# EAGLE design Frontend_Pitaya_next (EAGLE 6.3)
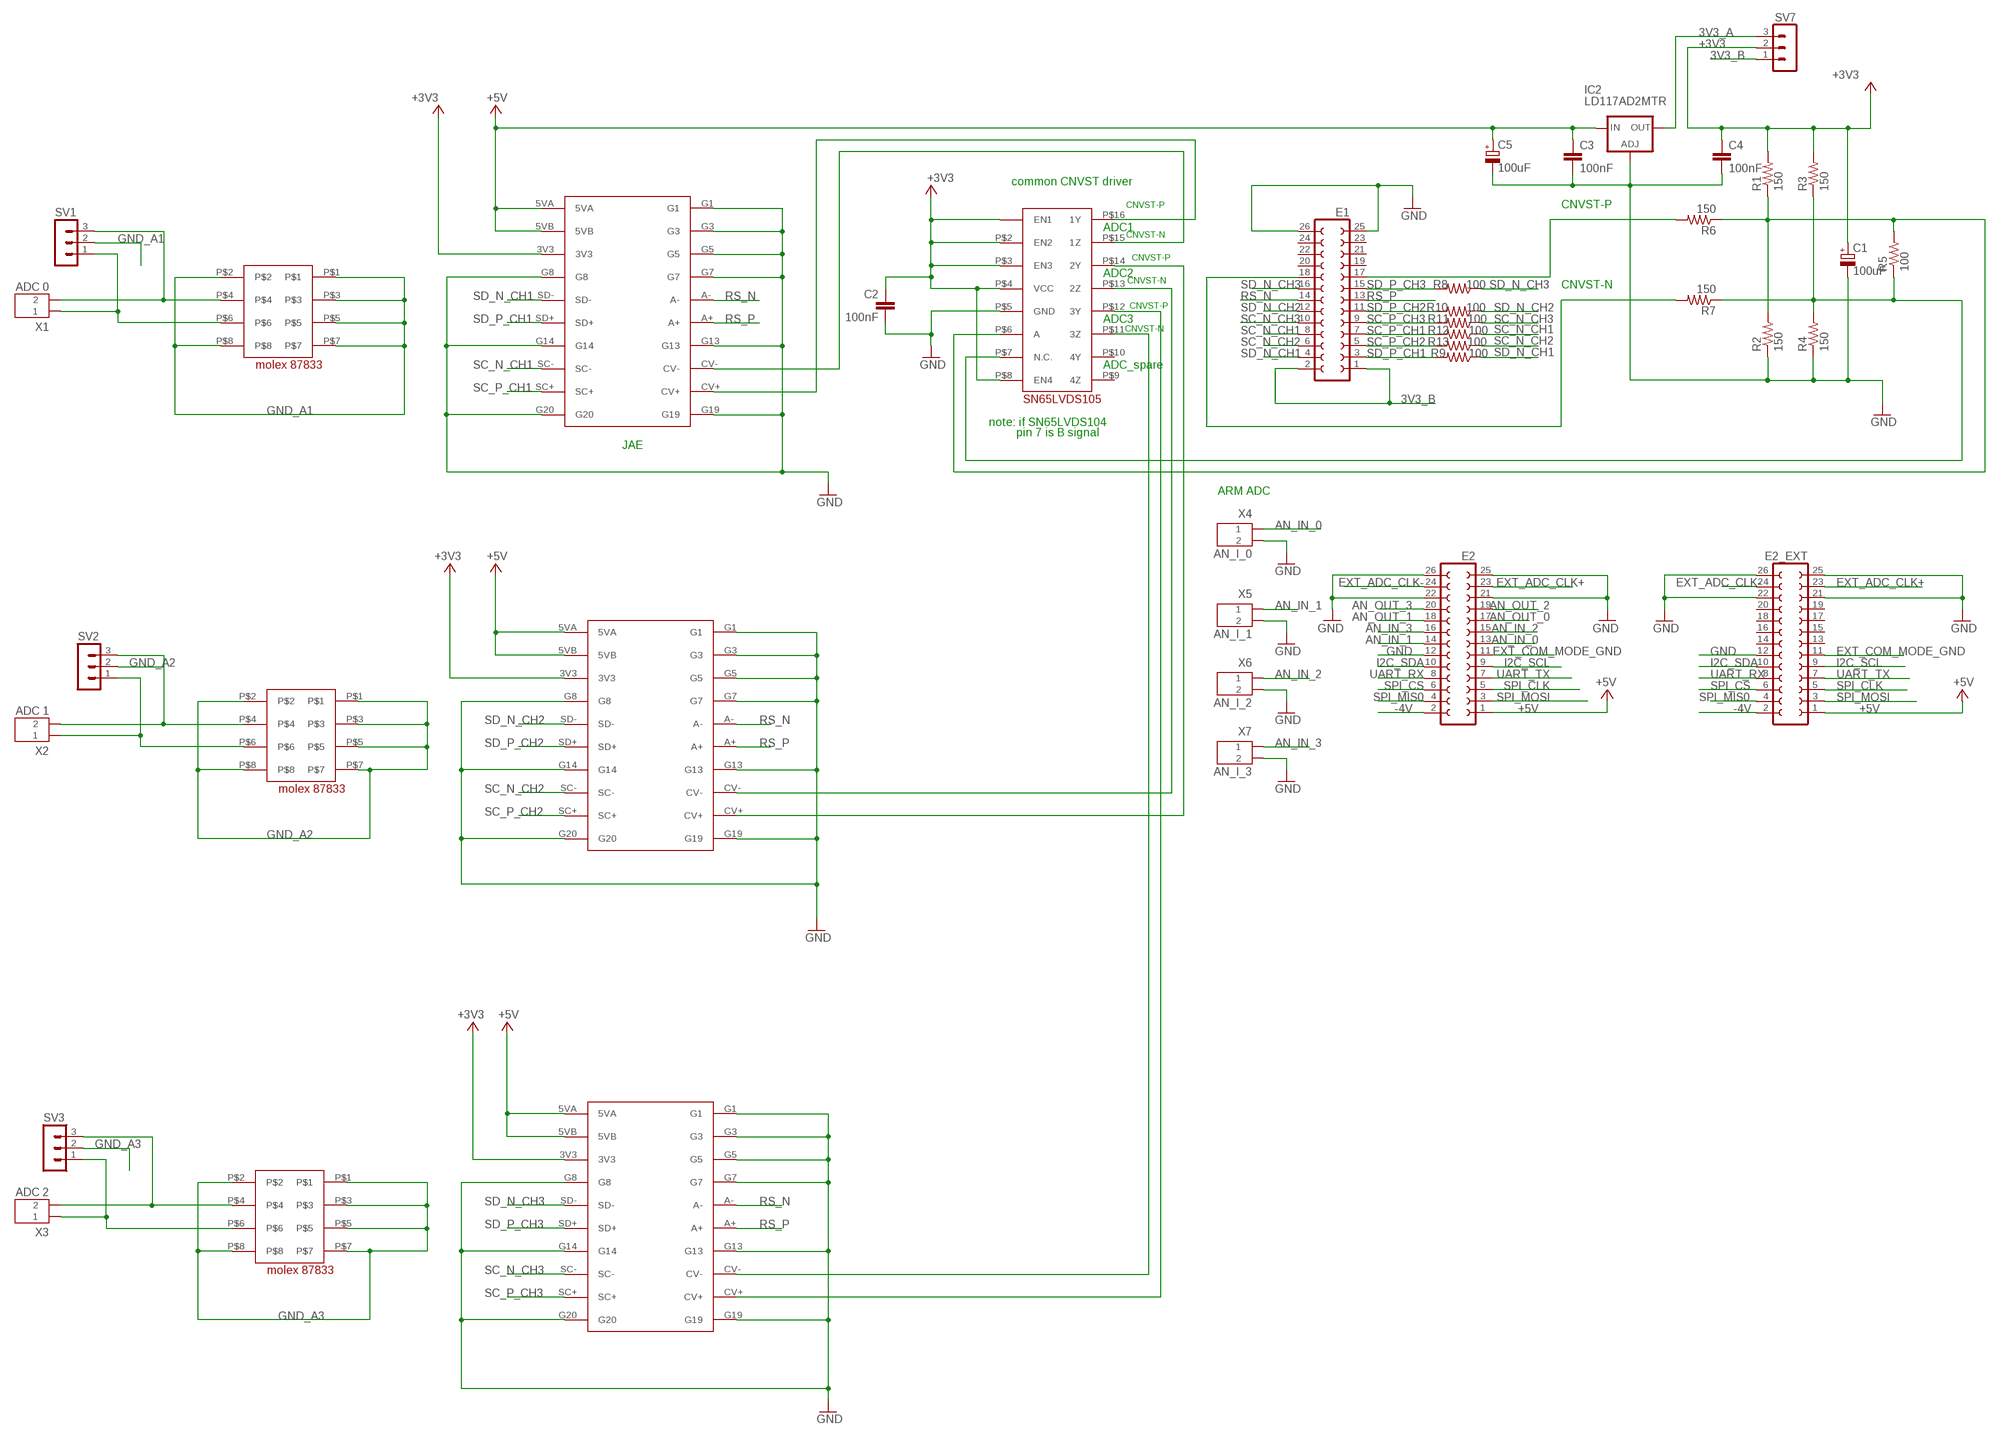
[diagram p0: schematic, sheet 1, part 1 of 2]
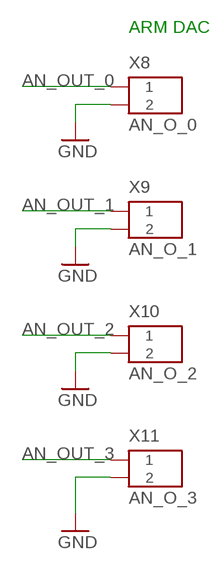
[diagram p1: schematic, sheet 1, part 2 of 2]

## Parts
C1  100uF  CPOL-EU085CS-1AR  [085CS_1AR]
C2  100nF  C-EUC0805  [C0805]
C3  100nF  C-EUC0805  [C0805]
C4  100nF  C-EUC0805  [C0805]
C5  100uF  CPOL-EU085CS-1AR  [085CS_1AR]
E1  FE13-2  [FE13-2]
E2  FE13-2  [FE13-2]
E2_EXT  FE13-2  [FE13-2]
IC2  LD117AD2MTR  [D2PACK]
R1  150  R-US_R0805  [R0805]
R2  150  R-US_R0805  [R0805]
R3  150  R-US_R0805  [R0805]
R4  150  R-US_R0805  [R0805]
R5  100  R-US_R0805  [R0805]
R6  150  R-US_R0805  [R0805]
R7  150  R-US_R0805  [R0805]
R8  100  R-US_R0805  [R0805]
R9  100  R-US_R0805  [R0805]
R10  100  R-US_R0805  [R0805]
R11  100  R-US_R0805  [R0805]
R12  100  R-US_R0805  [R0805]
R13  100  R-US_R0805  [R0805]
SV1  MA03-1  [MA03-1]
SV2  MA03-1  [MA03-1]
SV3  MA03-1  [MA03-1]
SV7  MA03-1  [MA03-1]
U$1  JAE_NEXT  [JAE_NEXT]
U$2  MOLEX87833_NEXT  [MOLEX87833NEXT]
U$3  SN65LVDS105  [SN65LVDS105]
U$4  MOLEX87833_NEXT  [MOLEX87833NEXT]
U$5  JAE_NEXT  [JAE_NEXT]
U$6  MOLEX87833_NEXT  [MOLEX87833NEXT]
U$7  JAE_NEXT  [JAE_NEXT]
X1  ADC 0  EZG-00-302  [EZG-00-302]
X2  ADC 1  EZG-00-302  [EZG-00-302]
X3  ADC 2  EZG-00-302  [EZG-00-302]
X4  AN_I_0  EZG-00-302  [EZG-00-302]
X5  AN_I_1  EZG-00-302  [EZG-00-302]
X6  AN_I_2  EZG-00-302  [EZG-00-302]
X7  AN_I_3  EZG-00-302  [EZG-00-302]
X8  AN_O_0  EZG-00-302  [EZG-00-302]
X9  AN_O_1  EZG-00-302  [EZG-00-302]
X10  AN_O_2  EZG-00-302  [EZG-00-302]
X11  AN_O_3  EZG-00-302  [EZG-00-302]

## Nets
3V3_A: IC2.2(OUT) SV7.3
3V3_B: E1.1 E1.2 SV7.1
+3V3: C1.+ C2.1 C4.1 R1.2 R3.2 SV7.2 U$1.3V3 U$3.P$1(EN1) U$3.P$2(EN2) U$3.P$3(EN3) U$3.P$4(VCC) U$3.P$8(EN4) U$5.3V3 U$7.3V3
+5V: C3.1 C5.+ E2.1 E2_EXT.1 IC2.3(IN) U$1.5VA U$1.5VB U$5.5VA U$5.5VB U$7.5VA U$7.5VB
-4V: E2.2 E2_EXT.2
AN_IN_0: E2.13 X4.1
AN_IN_1: E2.14 X5.1
AN_IN_2: E2.15 X6.1
AN_IN_3: E2.16 X7.1
AN_OUT_0: E2.17 X8.1
AN_OUT_1: E2.18 X9.1
AN_OUT_2: E2.19 X10.1
AN_OUT_3: E2.20 X11.1
EXT_ADC_CLK+: E2.23 E2_EXT.23
EXT_ADC_CLK-: E2.24 E2_EXT.24
EXT_COM_MODE_GND: E2.11 E2_EXT.11
GND: C1.- C2.2 C3.2 C4.2 C5.- E1.25 E1.26 E2.12 E2.21 E2.22 E2.25 E2.26 E2_EXT.12 E2_EXT.21 E2_EXT.22 E2_EXT.25 E2_EXT.26 IC2.1(ADJ) R2.1 R4.1 U$1.G1 U$1.G3 U$1.G5 U$1.G7 U$1.G8 U$1.G13 U$1.G14 U$1.G19 U$1.G20 U$3.P$5(GND) U$5.G1 U$5.G3 U$5.G5 U$5.G7 U$5.G8 U$5.G13 U$5.G14 U$5.G19 U$5.G20 U$7.G1 U$7.G3 U$7.G5 U$7.G7 U$7.G8 U$7.G13 U$7.G14 U$7.G19 U$7.G20 X4.2 X5.2 X6.2 X7.2 X8.2 X9.2 X10.2 X11.2
GND_A1: SV1.2 U$6.P$1 U$6.P$2 U$6.P$3 U$6.P$5 U$6.P$7 U$6.P$8
GND_A2: SV2.2 U$4.P$1 U$4.P$2 U$4.P$3 U$4.P$5 U$4.P$7 U$4.P$8
GND_A3: SV3.2 U$2.P$1 U$2.P$2 U$2.P$3 U$2.P$5 U$2.P$7 U$2.P$8
I2C_SCL: E2.9 E2_EXT.9
I2C_SDA: E2.10 E2_EXT.10
N$1: SV1.3 U$6.P$4 X1.2
N$9: E1.17 R6.2
N$11: E1.18 R7.2
N$24: SV1.1 U$6.P$6 X1.1
N$27: SV2.3 U$4.P$4 X2.2
N$30: U$3.P$16(1Y) U$7.CV+
N$31: U$3.P$15(1Z) U$7.CV-
N$32: SV2.1 U$4.P$6 X2.1
N$33: SV3.3 U$2.P$4 X3.2
N$34: R3.1 R4.2 R5.1 R7.1 U$3.P$7(N.C.)
N$35: U$3.P$14(2Y) U$5.CV+
N$36: SV3.1 U$2.P$6 X3.1
N$37: U$3.P$13(2Z) U$5.CV-
N$38: U$1.CV+ U$3.P$12(3Y)
N$39: U$1.CV- U$3.P$11(3Z)
N$40: R1.1 R2.2 R5.2 R6.1 U$3.P$6(A)
RS_N: E1.14 U$1.A- U$5.A- U$7.A-
RS_P: E1.13 U$1.A+ U$5.A+ U$7.A+
SC_N_CH1: E1.8 R12.1 U$7.SC-
SC_N_CH2: E1.6 R13.1 U$5.SC-
SC_N_CH3: E1.10 R11.1 U$1.SC-
SC_P_CH1: E1.7 R12.2 U$7.SC+
SC_P_CH2: E1.5 R13.2 U$5.SC+
SC_P_CH3: E1.9 R11.2 U$1.SC+
SD_N_CH1: E1.4 R9.1 U$7.SD-
SD_N_CH2: E1.12 R10.1 U$5.SD-
SD_N_CH3: E1.16 R8.1 U$1.SD-
SD_P_CH1: E1.3 R9.2 U$7.SD+
SD_P_CH2: E1.11 R10.2 U$5.SD+
SD_P_CH3: E1.15 R8.2 U$1.SD+
SPI_CLK: E2.5 E2_EXT.5
SPI_CS: E2.6 E2_EXT.6
SPI_MIS0: E2.4 E2_EXT.4
SPI_MOSI: E2.3 E2_EXT.3
UART_RX: E2.8 E2_EXT.8
UART_TX: E2.7 E2_EXT.7
Unconnected: E1.19 E1.20 E1.21 E1.22 E1.23 E1.24 E2_EXT.13 E2_EXT.14 E2_EXT.15 E2_EXT.16 E2_EXT.17 E2_EXT.18 E2_EXT.19 E2_EXT.20 U$3.P$9(4Z) U$3.P$10(4Y)

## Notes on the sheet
- common CNVST driver
- CNVST-P | CNVST-P
- ADC1
- CNVST-N
- CNVST-P
- ADC2
- CNVST-N
- CNVST-N
- CNVST-P
- ADC3
- CNVST-N
- ADC_spare
- note: if SN65LVDS104
- pin 7 is B signal
- JAE
- ARM DAC
- ARM ADC

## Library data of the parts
C1 C5 = resistor:CPOL-EU: POLARIZED CAPACITOR, European symbol
C2-C4 = resistor:C-EU: CAPACITOR, European symbol
E1 E2 E2_EXT = con-lsta:FE13-2: FEMALE HEADER; OC_FARNELL: unknown; OC_NEWARK: unknown
IC2 = v-reg:LD117A?*: Low drop fixed and adjustable positive voltage regulators 1 A Source: http://www.st.com/stonline/products/literature/ds/7194/ld1117axx.pdf
R1-R13 = resistor:R-US_: RESISTOR, American symbol
SV1-SV3 SV7 = con-lstb:MA03-1: PIN HEADER; OC_FARNELL: unknown; OC_NEWARK: unknown
U$1 U$5 U$7 = JAE_pad_extend:JAE_NEXT: JAE_Connector Next
U$2 U$4 U$6 = molex 87833 next:MOLEX87833_NEXT: Molex 87833 next
U$3 = SN65LVDS105:SN65LVDS105
X1-X11 = con-lemo:EZG-?-302: LEMO Connector; OC_FARNELL: unknown; OC_NEWARK: unknown

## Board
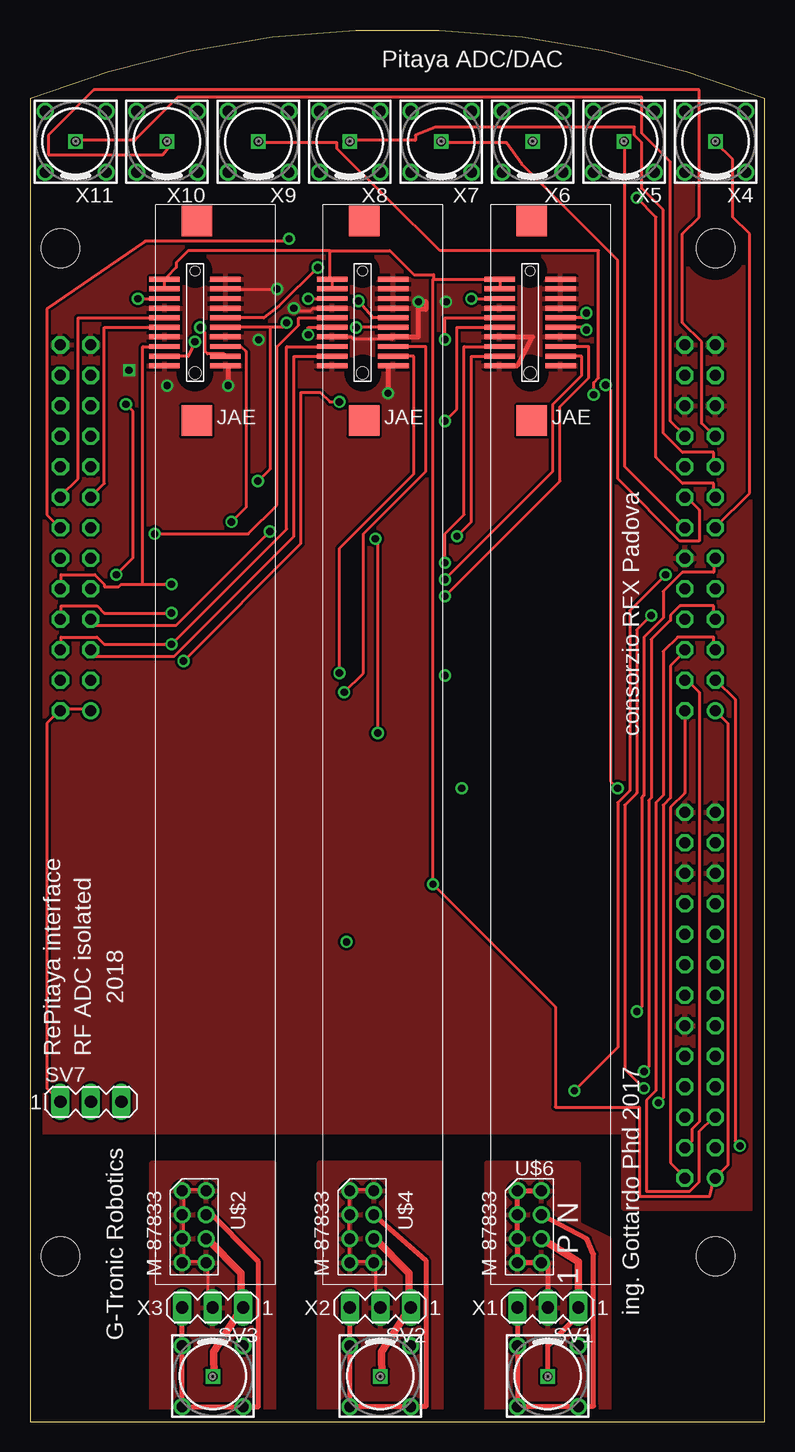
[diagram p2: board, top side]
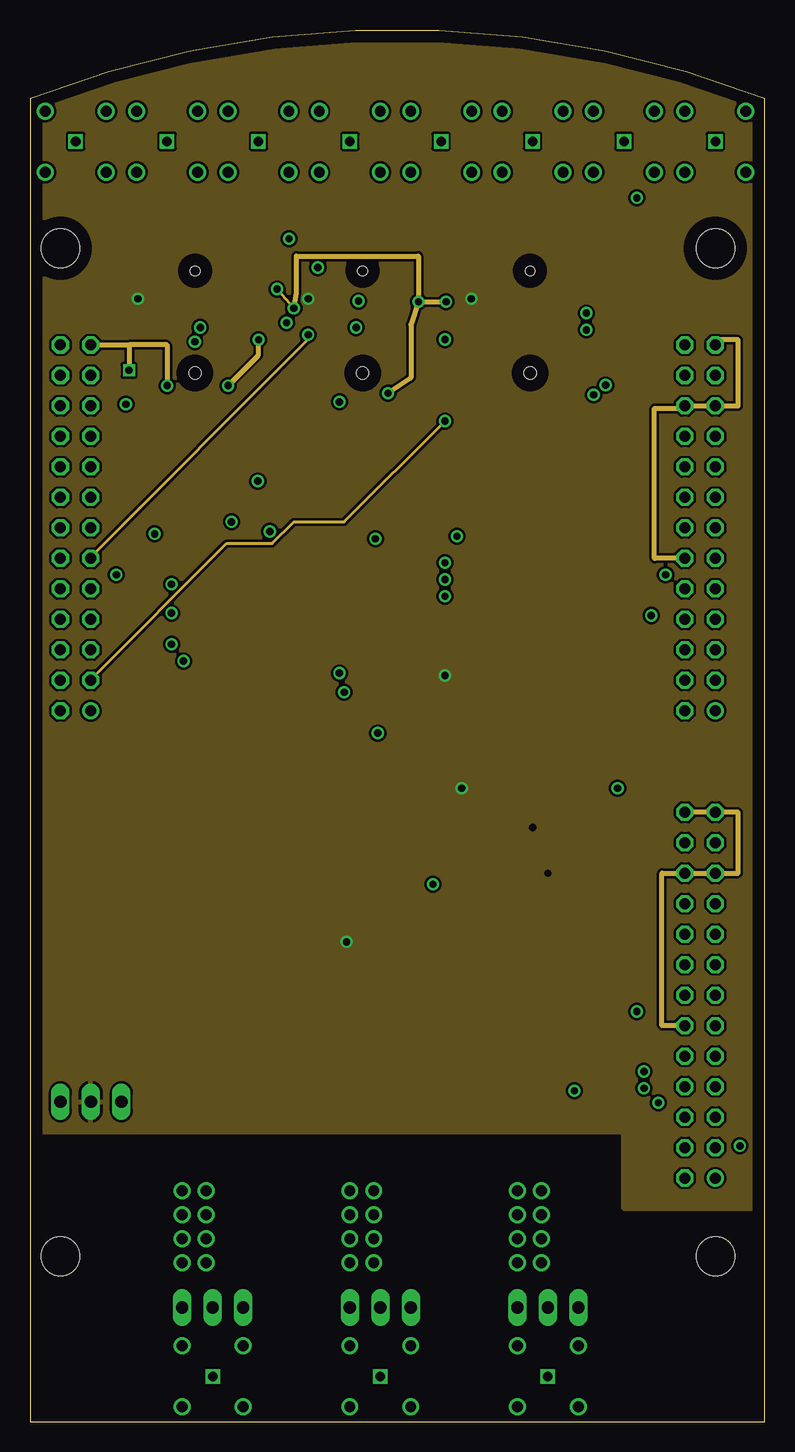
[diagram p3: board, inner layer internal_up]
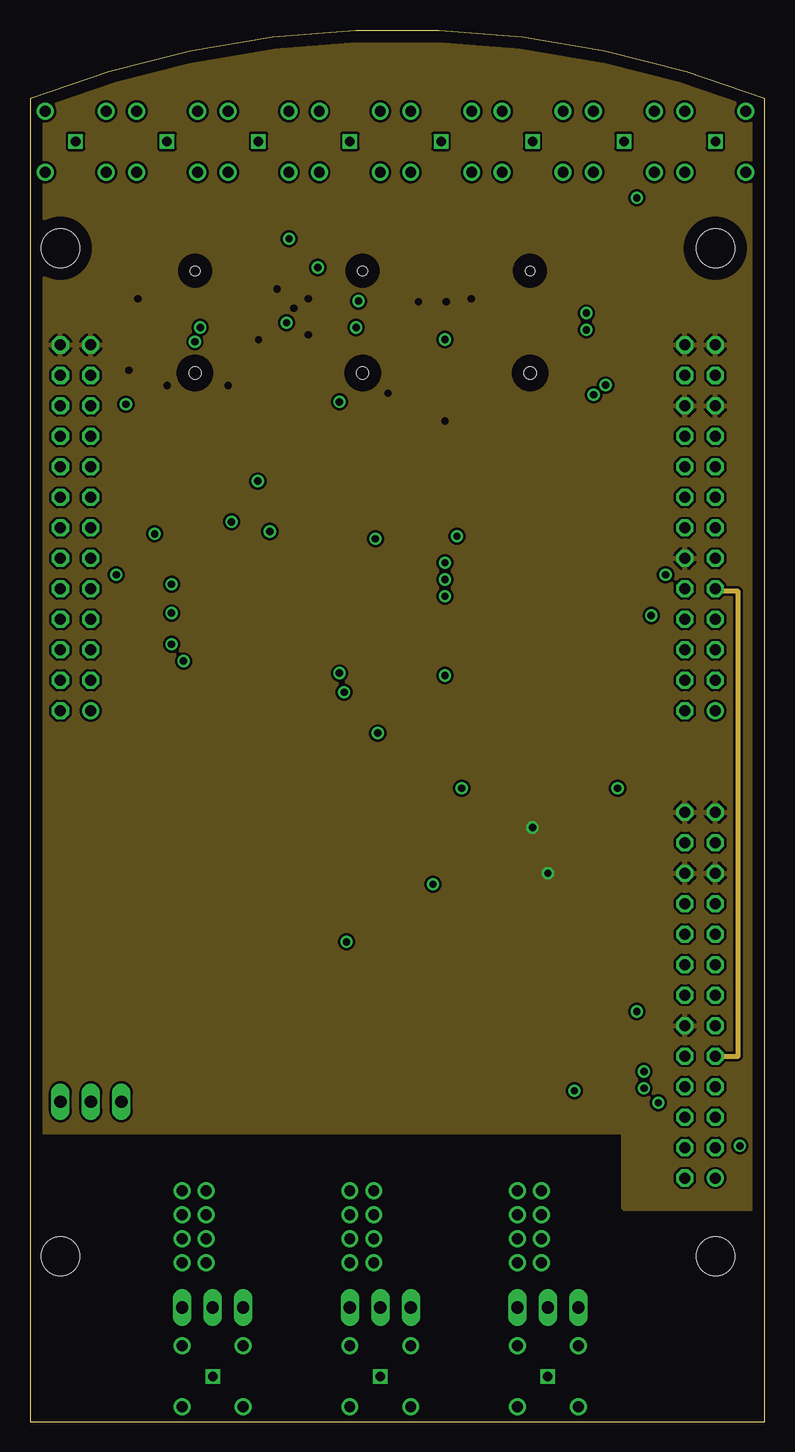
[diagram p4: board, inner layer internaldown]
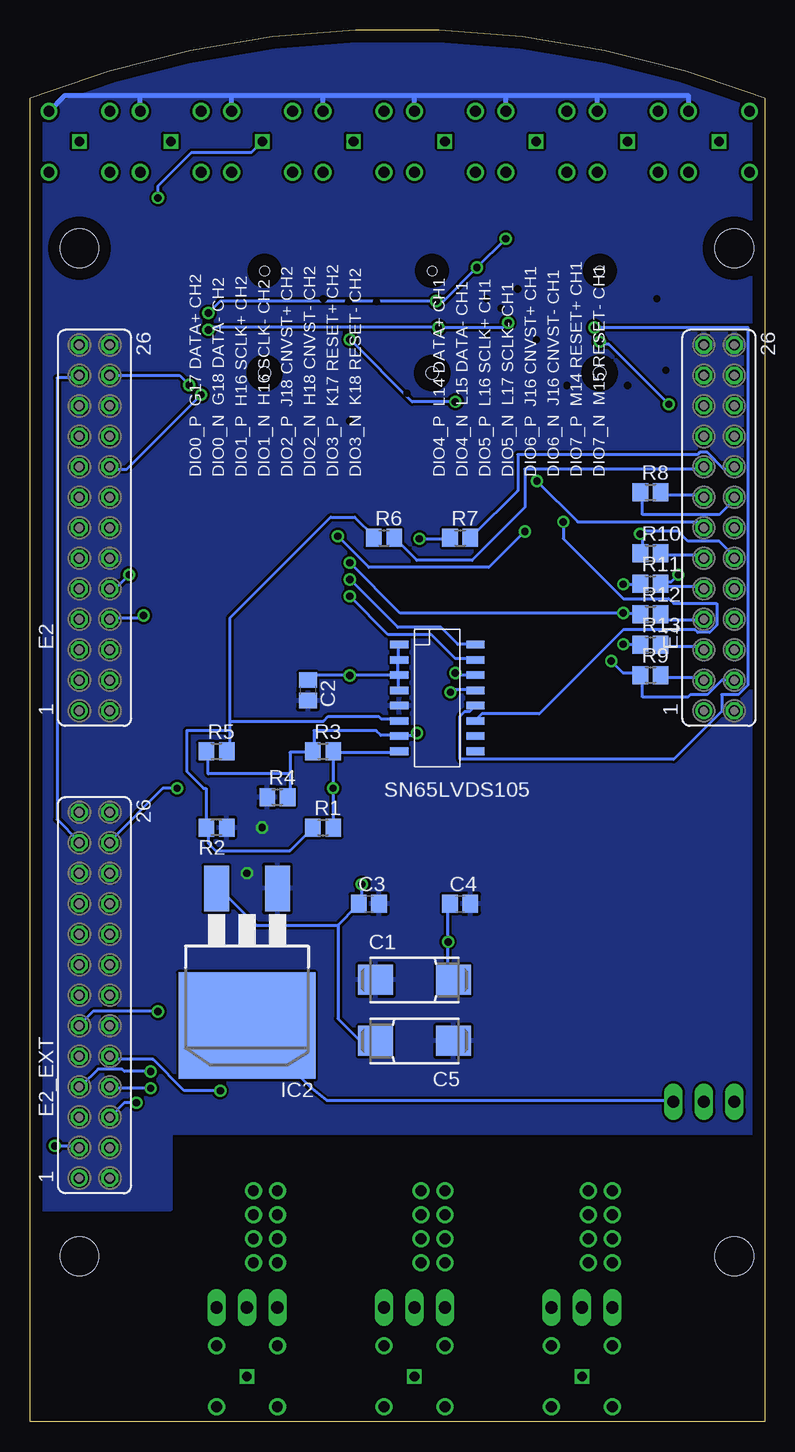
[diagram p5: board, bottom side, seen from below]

Size 61.27 x 115.99 mm. Coordinates in mm from the lower left corner, seen from the top.
Outline: 0,0 61.27,0 61.27,110.32 arc42 0,110.32 0,0
Copper layers ((1*2)+(15*16)): Top 0.035mm / dielectric 1.5mm / internal_up 0.035mm / dielectric 0.15mm / internaldown 0.035mm / dielectric 0.2mm / Bottom 0.035mm
Design rules "default *": minimum track width 10mil, minimum drill 24mil, track to track 8mil, track to pad 8mil, pad to pad 8mil, via to via 8mil, smd to smd 8mil, copper to edge 40mil, drill to drill 8mil, minimum pad ring 10mil, minimum via ring 8mil, stop-mask expansion 4mil, vias tented up to drill 0mil, thermal gap 10mil
Holes 3.2 mm at 2.54,97.8 57.15,97.8 2.54,13.8 57.15,13.8

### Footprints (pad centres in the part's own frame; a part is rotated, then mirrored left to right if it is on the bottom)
085CS_1AR = smd 2.9 x 2.5: + 3.25,0; - -3.25,0
C0805 = smd 1.3 x 1.5: 1 -0.85,0; 2 0.85,0
FE13-2 = drill 0.914: 1 -15.24,1.27 | drill 0.914 octagon: 2 -15.24,-1.27; 3 -12.7,1.27; 4 -12.7,-1.27; 5 -10.16,1.27; 6 -10.16,-1.27; 7 -7.62,1.27; 8 -7.62,-1.27; 9 -5.08,1.27; 10 -5.08,-1.27; 11 -2.54,1.27; 12 -2.54,-1.27; 13 0,1.27; 14 0,-1.27; 15 2.54,1.27; 16 2.54,-1.27; 17 5.08,1.27; 18 5.08,-1.27; 19 7.62,1.27; 20 7.62,-1.27; 21 10.16,1.27; 22 10.16,-1.27; 23 12.7,1.27; 24 12.7,-1.27; 25 15.24,1.27; 26 15.24,-1.27
D2PACK = smd 2.083 x 3.81: 1 -2.54,-8.89; 3 2.54,-8.89 | smd 11.43 x 8.89: 2 0,2.54
R0805 = smd 1.3 x 1.5: 1 -0.85,0; 2 0.85,0
MA03-1 = drill 1.016 long: 1 -2.54,0; 2 0,0; 3 2.54,0
JAE_NEXT = smd 2.54 x 0.406: 3V3 -2.748,1.155; 5VA -2.748,2.755; 5VB -2.748,1.955; A+ 2.337,-1.245; A- 2.337,-0.445; CV+ 2.337,-3.645; CV- 2.337,-2.845; G1 2.337,2.755; G3 2.337,1.955; G5 2.337,1.155; G7 2.337,0.355; G8 -2.748,0.355; G13 2.337,-2.045; G14 -2.748,-2.045; G19 2.337,-4.445; G20 -2.748,-4.445; SC+ -2.748,-3.645; SC- -2.748,-2.845; SD+ -2.748,-1.245; SD- -2.748,-0.445 | smd 2.54 x 2.54: P$1 -0.071,7.62; P$2 -0.071,-9.017 | hole 0.8: -0.205,3.455 | hole 1: -0.205,-5.045
MOLEX87833NEXT = drill 0.9: P$1 -1.27,1.27; P$2 -1.27,3.27; P$3 0.73,1.27; P$4 0.73,3.27; P$5 2.73,1.27; P$6 2.73,3.27; P$7 4.73,1.27; P$8 4.73,3.27
SN65LVDS105 = smd 1.524 x 0.635: P$1 -2.54,8.89; P$2 -2.54,7.62; P$3 -2.54,6.35; P$4 -2.54,5.08; P$5 -2.54,3.81; P$6 -2.54,2.54; P$7 -2.54,1.27; P$8 -2.54,0; P$9 3.81,0; P$10 3.81,1.27; P$11 3.81,2.54; P$12 3.81,3.81; P$13 3.81,5.08; P$14 3.81,6.35; P$15 3.81,7.62; P$16 3.81,8.89
EZG-00-302 = drill 0.6 pad 1: 1 0,-0.035; 2 -2.54,-2.505 | drill 0.9 pad 1.2: M1 -2.54,2.54; M2 2.54,2.54; M3 2.54,-2.54; M4 -2.54,-2.54

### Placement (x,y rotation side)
C1  29.21,36.83 0 bottom
C2  38.1,60.96 270 bottom
C3  33.02,43.18 0 bottom
C4  25.4,43.18 0 bottom
C5  29.21,31.75 180 bottom
E1  3.81,74.5 90 bottom
E2  55.88,74.5 90 bottom
E2_EXT  55.88,35.56 90 bottom
IC2  43.18,35.56 180 bottom
R1  36.83,49.53 0 bottom
R2  45.72,49.53 180 bottom
R3  36.83,55.88 0 bottom
R4  40.64,52.07 0 bottom
R5  45.72,55.88 0 bottom
R6  31.75,73.66 0 bottom
R7  25.4,73.66 0 bottom
R8  9.53,77.47 0 bottom
R9  9.53,62.23 0 bottom
R10  9.53,72.39 0 bottom
R11  9.53,69.85 0 bottom
R12  9.53,67.31 0 bottom
R13  9.53,64.77 0 bottom
SV1  43.18,9.53 180 top
SV2  29.21,9.53 180 top
SV3  15.24,9.53 180 top
SV7  5.08,26.67 0 top
U$1  13.97,92.46 0 top
U$2  11.43,18 270 top
U$3  27.94,55.88 0 bottom
U$4  25.4,18 270 top
U$5  27.94,92.46 0 top
U$6  39.37,18 270 top
U$7  41.91,92.46 0 top
X1  43.18,3.81 0 top
X2  29.21,3.81 0 top
X3  15.24,3.81 0 top
X4  57.15,106.68 180 top
X5  49.53,106.68 180 top
X6  41.91,106.68 180 top
X7  34.29,106.68 180 top
X8  26.67,106.68 180 top
X9  19.05,106.68 180 top
X10  11.43,106.68 180 top
X11  3.81,106.68 180 top

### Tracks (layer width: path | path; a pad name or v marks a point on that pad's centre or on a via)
3V3_A
  Bottom 0.254: SV7.3 7.8,26.8 36.53,26.8 37.8,27.8 43,33 IC2.2
3V3_B
  Top 0.254: E1.1 5,59.4 2.6,59.4 E1.2 2.4,59.2 1.4,58.2 1.4,27.8 2.4,26.8 SV7.1
+3V3  (via drill 0.61, 0.61 layers 1-2)
  Top 0.254: v9,93.6 11.2,93.6 U$1.3V3 | v23.2,93.6 25,93.6 U$5.3V3 | v36.8,93.6 39,93.6 U$7.3V3
  Bottom 0.254: R1.2 36,49.6 v36,52.8 36,55.8 R3.2 35.8,55.8 30.6,55.8 U$3.P$8 | U$3.P$1 30.6,64.6 30.6,63.6 U$3.P$2 30.6,63.4 30.6,62.4 U$3.P$3 30.6,62.2 | 30.6,62.2 v34.6,62.2 37.8,62.2 38,62 C2.1 | 30.6,62.2 30.6,61 U$3.P$4 | C4.1 26.4,43 v26.4,40 26.4,37 26,37 C1.+
  pour internal_up: -11.43,121.92 69.85,121.92 69.85,17.78 49.53,17.78 49.53,24.13 -11.43,24.13
+5V  (via drill 0.61)
  Top 0.254: E2.1 57.2,59.2 58.2,58.2 58.2,21.4 57.2,20.4 E2_EXT.1 57,20.2 56.67,18.8 50.8,18.8 50.8,26.22 43.8,26.22 43.8,34.6 v33.6,44.8 33.6,95.2 33.66,95.2 | U$7.5VB 39.2,94.6 39.2,95.2 U$7.5VA 39,95.2 33.66,95.2 | U$1.5VB 11.2,94.6 11.2,95.2 U$1.5VA 11.4,95.4 12.2,96.2 12.2,96.6 13.2,97.6 25,97.6 | U$5.5VB 25.2,94.6 U$5.5VA 25,95.4 25,97.6 | 33.66,95.2 33.66,95.6 32,95.6 30,97.6 25,97.6
  Bottom 0.254: 35.6,41.4 34,43 C3.1 33.8,43.2 33.6,43.2 v33.6,44.8 | 35.6,41.4 42.4,41.4 45.4,44.4 45.6,44.4 IC2.3 | 35.6,41.4 35.6,33.61 33.87,31.88 C5.+
-4V
  Top 0.254: E2_EXT.2 54.6,20.4 53.4,21.6 53.4,51.2 54.6,52.4 54.6,59.2 E2.2
AN_IN_0
  Top 0.254: X4.1 57.2,106.6 58.6,105.2 58.6,100.4 60,99 60,77.4 57.2,74.6 E2.13
AN_IN_1
  Top 0.254: X5.1 49.6,106.6 49.6,79.6 54.6,74.6 E2.14
AN_IN_2  (via drill 0.61)
  Top 0.254: v50.6,102 52.2,100.4 52.2,80.4 54.4,78.2 57,78.2 57,77.2 E2.15
  Bottom 0.254: v50.6,102 50.6,103 47.8,105.8 42.8,105.8 42,106.6 X6.1
AN_IN_3
  Top 0.254: X7.1 34.4,106.6 39.73,106.6 41,104.8 49,96.8 49,78.6 54.2,73.4 55.8,73.4 55.8,76 54.8,77 E2.16
AN_OUT_0
  Top 0.254: X8.1 26.8,106.8 32.13,106.8 32.13,107.2 33.8,107.9 50.4,107.9 50.4,107.2 51,106.6 51,102.8 52.8,101 52.8,82.4 54.4,80.8 57,80.8 57,79.6 E2.17
AN_OUT_1  (via drill 0.61)
  Top 0.254: v47,85.6 47,86.6 47.4,87 47.4,97.6 34.2,97.6 25.6,106.1 25.6,106.6 19.2,106.6 X9.1
  Bottom 0.254: v47,85.6 53.2,79.4 54.6,79.4 E2.18
AN_OUT_2
  Top 0.254: X10.1 11.4,106.6 11.87,106.6 11.07,105.6 1.53,105.6 1.53,107.2 5.33,111 55.8,111 55.8,100.4 54.4,99 54.4,91.6 56,90 56,83.2 57,82.2 E2.19
AN_OUT_3
  Top 0.254: X11.1 4,106.8 8.73,106.8 12.33,110.4 51,110.4 51,107.4 53.4,105 53.4,83.4 54.6,82.2 E2.20
EXT_ADC_CLK+
  Bottom 0.254: E2_EXT.23 57.2,48.4 59,50.2 59,87 57.4,87 57.2,87.2 E2.23
EXT_ADC_CLK-  (via drill 0.61)
  Top 0.254: v49,52.8 48.4,53.4 48.4,86 v48,86.4
  Bottom 0.254: v49,52.8 50.2,52.8 54.6,48.4 E2_EXT.24 | v48,86.4 48.8,87.2 E2.24
EXT_COM_MODE_GND  (via drill 0.61)
  Top 0.254: v50.6,34.2 51,34.6 51,52 51.2,52.2 51.2,65.4 52.8,67 52.8,69.2 54.4,70.8 57,70.8 57,71.8 E2.11
  Bottom 0.254: v50.6,34.2 56,34.2 57,33.2 E2_EXT.11
GND  (via drill 0.6 layers 1-2, 0.6 layers 15-16, 0.61 layers 1-2)
  Top 0.254: U$5.G14 26.8,90.4 27,90.2 30.2,90.2 30.2,90.4 U$5.G13 | v22,92.8 22,92.6 23.4,92.6 23.6,92.8 25,92.8 U$5.G8 | v20.6,94.4 16.4,94.4 U$1.G3
  Top 0.406: U$5.G19 29.84,88.01 v29.84,85.72 | U$5.G13 32.38,90.41 v32.38,93.34 | v32.38,93.34 33.02,93.34 33.02,92.71 32.38,92.71 v32.38,93.34 | U$7.G14 41.91,90.41 40.64,88.01 U$7.G20 | U$1.G19 16.51,88.01 v16.51,86.36
  internal_up 0.254: v20.6,94.4 v22,92.8 | 34.8,93.2 v34.7,93.34
  internal_up 0.406: E2.12 52.07,71.96 52.07,84.45 54.61,84.45 E2.22 E2.21 59.05,84.66 59.05,90.17 57.15,90.17 E2.25 | E2_EXT.12 52.7,33.02 52.7,45.72 E2_EXT.22 E2_EXT.21 59.05,45.72 59.05,50.8 E2_EXT.25 E2_EXT.26 | E1.25 8.26,89.74 | v11.43,86.36 11.43,89.74 8.26,89.74 | v32.38,93.34 v34.7,93.34 | v32.38,93.34 31.75,91.44 31.75,87 v29.84,85.72 | 22.02,92.81 22.23,94.08 22.23,97.16 32.38,97.16 v32.38,93.34 | 8.26,89.74 v8.26,87.63 | v16.51,86.36 19.05,88.9 v19.05,90.17
  Bottom 0.406: X11.2 6.35,110.49 13.97,110.49 | X10.2 13.97,110.49 | 13.97,110.49 21.59,110.49 | X9.2 21.59,110.49 | 21.59,110.49 29.21,110.49 | X8.2 29.21,110.49 | 29.21,110.49 36.83,110.49 | X7.2 36.83,110.49 | 36.83,110.49 44.45,110.49 | X6.2 44.45,110.49 | 44.45,110.49 52.07,110.49 | X5.2 52.07,110.49 | 52.07,110.49 58.42,110.49 X4.2
  other vias: 41.91,49.53 43.18,45.72
  pour Bottom: -6.35,118.11 64.77,118.11 64.77,17.78 49.53,17.78 49.53,24.13 -6.35,24.13
  pour Top: -8.89,119.38 67.31,119.38 68.58,17.78 49.53,17.78 49.53,24.13 -7.62,24.13
  pour internaldown: -12.7,123.19 73.66,123.19 73.66,17.78 49.53,17.78 49.53,24.13 -12.7,24.13
GND_A1
  Top 0.406: SV1.2 43.18,13.27 U$6.P$8 U$6.P$7 U$6.P$5 U$6.P$3 U$6.P$1 U$6.P$2
  pour Top: 38.1,21.59 45.72,21.59 45.72,16.51 48.26,15.24 48.26,-1.27 38.1,-1.27
GND_A2
  Top 0.254: U$4.P$2 28.6,19.4 26.8,19.4 U$4.P$1 26.6,19.2 26.6,17.4 U$4.P$3 26.6,17.2 26.6,15.4 U$4.P$5 26.6,15.2 26.6,13.4 U$4.P$7 26.8,13.4 28.6,13.4 U$4.P$8 28.8,13.2 28.8,10 29.2,9.6 SV2.2
  pour Top: 24.13,21.59 34.29,21.59 34.29,-1.27 24.13,-1.27
GND_A3
  Top 0.254: U$2.P$2 14.6,19.4 12.8,19.4 U$2.P$1 12.8,19.2 12.8,17.4 U$2.P$3 12.8,17.2 12.8,15.4 U$2.P$5 12.8,15.2 12.8,13.4 | 12.8,13.4 14.6,13.4 U$2.P$8 14.8,13.2 14.8,10 15.2,9.6 SV3.2 | 12.8,13.4 U$2.P$7
  pour Top: 10.16,21.59 20.32,21.59 20.32,-1.27 10.16,-1.27
I2C_SCL
  internaldown 0.406: E2_EXT.9 59.05,30.48 59.05,69.22 57.15,69.22 E2.9
I2C_SDA  (via drill 0.61)
  Top 0.254: v45.4,27.6 49,31.2 49,51.6 50,52.6 50,67.6 v53,70.6
  Bottom 0.254: v45.4,27.6 48.4,27.6 51,30.2 54.4,30.2 54.6,30.4 E2_EXT.10 | v53,70.6 54,69.6 54.6,69.6 E2.10
N$1
  Top 0.406: SV1.3 X1.2 | 40.64,1.27 X1.2 | X1.2 46.99,1.3 46.99,13.97 46.45,15.24 U$6.P$4
N$2  (via drill 0.8)
  other vias: 29.21,3.78
N$3  (via drill 0.8)
  other vias: 15.24,3.78
N$4  (via drill 0.8)
  other vias: 3.81,106.7
N$5  (via drill 0.8)
  other vias: 11.43,106.7
N$6  (via drill 0.8)
  other vias: 19.05,106.7
N$7  (via drill 0.8)
  other vias: 26.67,106.7
N$8  (via drill 0.8)
  other vias: 34.29,106.7
N$9
  Bottom 0.254: R6.2 30.8,73.6 29,71.8 24.4,71.8 20,76.2 20,79.4 5.2,79.4 E1.17
N$10  (via drill 0.8)
  other vias: 41.91,106.7
N$11
  Bottom 0.254: R7.2 24.4,73.8 20.6,77.6 20.6,80.6 5.6,80.6 5.4,80.8 4.8,80.8 3.4,79.4 2.6,79.4 E1.18
N$12  (via drill 0.8)
  other vias: 49.53,106.7
N$13  (via drill 0.8)
  other vias: 57.15,106.7
N$24  (via drill 0.8)
  Top 0.406: X1.1 v43.18,3.78 43.18,6.35 45.72,8.89 SV1.1 | 42.64,15.24 U$6.P$6
  Top 0.61: SV1.1 45.72,13.34 42.64,15.24
N$27
  Top 0.406: U$4.P$4 33.02,13.46 33.02,1.27 26.67,1.27 X2.2 SV2.3
N$30  (via drill 0.61)
  Top 0.254: v34.6,70.2 43.6,79.2 43.6,84.8 46,87.2 46,88.8 44.4,88.8 U$7.CV+
  Bottom 0.254: v34.6,70.2 30.6,66.2 27,66.2 25.6,64.8 24.2,64.8 U$3.P$16
N$31  (via drill 0.61)
  Top 0.254: v34.6,68.8 44.2,78.4 44.2,84.6 46.6,87 46.6,89.6 44.4,89.6 U$7.CV-
  Bottom 0.254: v34.6,68.8 31.4,65.6 27.8,65.6 25.8,63.6 24.2,63.6 U$3.P$15
N$32
  Top 0.254: 29.4,3.8 X2.1 | 31.6,9.4 SV2.1 31.6,9.6 | 28.8,15.2 U$4.P$6
  Top 0.61: 29.4,3.8 29.33,5 29.33,5.86 31.6,9.4 | 28.8,15.2 31.6,12.4 31.6,9.6
N$33
  Top 0.406: U$2.P$4 14.7,17.78 19.05,13.34 19.05,1.27 12.7,1.27 X3.2 SV3.3
N$34  (via drill 0.61)
  Top 0.254: v28.8,73.6 29,73.4 v29,57.4
  Bottom 0.254: 39.6,54 39.6,55.8 37.8,55.8 R3.1 37.6,56 37.6,57.6 32.4,57.6 32,57.2 30.6,57.2 U$3.P$7 30.4,57.2 29.2,57.2 v29,57.4 | 39.6,54 39.6,52.2 R4.2 | 39.6,54 46.4,54 46.4,55.8 R5.1 | v28.8,73.6 26.4,73.6 R7.1
N$35  (via drill 0.61)
  Top 0.254: v25.8,62.4 25.8,72.8 32,79 32,88.8 30.4,88.8 U$5.CV+
  Bottom 0.254: v25.8,62.4 25.6,62.2 24.2,62.2 U$3.P$14
N$36
  Top 0.254: 15.4,3.8 X3.1 | 17.6,9.4 SV3.1 17.6,9.6 | 14.8,15.2 U$2.P$6
  Top 0.61: 15.4,3.8 15.33,5 15.33,5.86 17.6,9.4 | 14.8,15.2 17.6,12.4 17.6,9.6
N$37  (via drill 0.61)
  Top 0.254: v26.2,60.8 27.8,62.4 27.8,74 33,79.2 33,89.6 30.4,89.6 U$5.CV-
  Bottom 0.254: v26.2,60.8 26,61 24.2,61 U$3.P$13
N$38  (via drill 0.61)
  Top 0.254: v14.2,91.2 14.6,90.8 14.6,89.2 14.8,89 16.2,89 U$1.CV+
  Bottom 0.254: v14.2,91.2 1.4,91.2 1.4,61.4 2.2,60.6 3.6,60.6 3.6,59.2 7.6,55.2 25.4,55.2 25.4,58.8 25,59.2 24.6,59.2 24.2,59.6 U$3.P$12
N$39  (via drill 0.61)
  Top 0.254: v16.8,75 18,76.2 18,89.2 17.6,89.6 16.4,89.6 U$1.CV-
  Bottom 0.254: v16.8,75 16.8,73.6 11.8,68.6 8,68.6 7.6,68.2 4,68.2 4,66.4 4.6,65.8 5.6,65.8 5.8,66 11.8,66 18.8,59 23.6,59 24,58.6 U$3.P$11
N$40
  Bottom 0.254: R1.1 37.8,49.4 39.6,47.6 45.8,47.6 46.4,48.2 46.4,49.4 R2.2 46.6,49.6 46.6,52.8 46.8,52.8 48.2,54.2 48.2,57.6 44.6,57.6 | 44.6,57.6 44.6,56 44.8,56 R5.2 | 44.6,57.6 44.6,58.4 | 44.6,58.4 44.6,67 36.2,75.4 34.2,75.4 32.6,73.8 R6.1 | 44.6,58.4 36.8,58.4 36.4,58.8 32.2,58.8 32,58.6 30.6,58.6 U$3.P$6
RS_N  (via drill 0.61)
  Top 0.254: v24,96.2 20.75,93 19.48,92 16.4,92 U$1.A- | v27.4,93.4 28.6,92 30.2,92 U$5.A- | v46.4,92.4 46.4,92 44.4,92 U$7.A- | v21.6,98.6 21.6,98.4 9.6,98.4 1.4,92.74 1.4,75.6 2.4,74.6 E1.14
  Bottom 0.254: v46.4,92.4 45.4,93.4 v27.4,93.4 26.8,93.4 v24,96.2 v21.6,98.6
RS_P  (via drill 0.61)
  Top 0.254: 20,91.2 21.4,91.2 v21.4,91.6 | 20,91.2 16.4,91.2 U$1.A+ | v27.2,91.2 30.2,91.2 U$5.A+ | v46.4,91 46.4,91.2 44.4,91.2 U$7.A+ | v19,78.4 20,79.4 20,91.2
  Bottom 0.254: v21.4,91.6 21.8,91.2 v27.2,91.2 46.2,91.2 v46.4,91 | v19,78.4 15.6,75 5.6,75 5.2,74.6 E1.13
SC_N_CH1  (via drill 0.61)
  Top 0.254: v11.8,67.4 6.2,67.4 5.6,68 2.6,68 2.6,67 E1.8 | v34.6,71.6 34.6,74 36.2,75.6 36.2,89.6 39,89.6 U$7.SC-
  Bottom 0.254: R12.1 10.4,67.4 v11.8,67.4 30.4,67.4 v34.6,71.6
SC_N_CH2  (via drill 0.61)
  Top 0.254: E1.6 2.6,64.4 2.6,65.4 5.6,65.4 6.2,64.8 v11.8,64.8 21.4,74.4 21.4,89.6 25,89.6 U$5.SC-
  Bottom 0.254: v11.8,64.8 10.4,64.8 R13.1
SC_N_CH3  (via drill 0.61)
  Top 0.254: 9.4,69.8 7.6,69.8 7.4,69.6 6.2,69.6 6.2,69.8 5.4,70.6 2.6,70.6 2.6,69.6 E1.10 | 9.4,69.8 v11.8,69.8 | 9.4,69.8 9.4,89.6 11.2,89.6 U$1.SC-
  Bottom 0.254: v11.8,69.8 10.4,69.8 R11.1
SC_P_CH1  (via drill 0.61)
  Top 0.254: v35.6,73.8 36.8,75 36.8,88.8 39,88.8 U$7.SC+ | v20,74.2 12.2,66.4 5.2,66.4 5.2,66.8 E1.7
  Bottom 0.254: R12.2 8.6,67.2 8.2,66.8 5.2,66.8 E1.7 | v35.6,73.8 33,71.2 23,71.2 v20,74.2
SC_P_CH2
  Top 0.254: U$5.SC+ 25,88.8 22,88.8 22,73.8 12,63.8 5.2,63.8 5.2,64.2 E1.5
  Bottom 0.254: R13.2 8.6,64.6 5.4,64.6 5.2,64.4 E1.5
SC_P_CH3  (via drill 0.6, 0.61)
  Top 0.254: v13.75,90 13.2,88.8 11.4,88.8 U$1.SC+ | v8,84.8 8.6,84.2 8.6,72 v7.2,70.6
  Bottom 0.254: E1.9 5.2,69.6 8.4,69.6 8.6,69.8 R11.2 8.6,70 7.8,70 v7.2,70.6 | v13.75,90 14,89.8 13,89.8 v8,84.8
SD_N_CH1  (via drill 0.61)
  Top 0.254: v34.6,90.2 34.6,92 39,92 U$7.SD- | v25.8,85 25,85 24.2,85.8 22.6,85.8 22.6,73.2 v12.8,63.4
  Bottom 0.254: E1.4 3.6,61.8 4.8,60.6 6.2,60.6 6.4,60.4 10.2,60.4 10.2,62.2 R9.1 10.4,62.4 11.8,62.4 v12.8,63.4 | v34.6,90.2 29.4,85 v25.8,85
SD_N_CH2  (via drill 0.61)
  Top 0.254: v10.4,74 18.2,74 20.6,76.4 20.6,89.6 22.4,91.4 22.4,92 25,92 U$5.SD-
  Bottom 0.254: 10.2,74 10.2,74.2 7.2,74.2 6.4,73.4 3.8,73.4 2.4,72 E1.12 | 10.2,74 10.2,72.4 R10.1 | 10.2,74 v10.4,74
SD_N_CH3
  Top 0.254: U$1.SD- 11.2,92 4,92 4,78.6 2.6,77.2 E1.16
  Bottom 0.254: R8.1 10.2,77.4 10.2,75.6 3.8,75.6 2.4,77 E1.16
SD_P_CH1  (via drill 0.61 layers 1-2)
  Top 0.254: v34.6,83.4 35.6,84.4 35.6,91.2 39,91.2 U$7.SD+
  internal_up 0.254: v34.6,83.4 26.2,75 22,75 20.2,73.2 16.4,73.2 5,61.8 E1.3
  Bottom 0.254: R9.2 8.6,62.2 8.4,62 5.4,62 5.2,61.8 E1.3
SD_P_CH2  (via drill 0.61 layers 1-2)
  Top 0.254: v23.2,90.6 23.2,91.2 25,91.2 U$5.SD+
  internal_up 0.254: v23.2,90.6 23.2,90.2 5,72 E1.11
  Bottom 0.254: R10.2 8.6,72.2 5.4,72.2 5.2,72 E1.11
SD_P_CH3
  Top 0.254: U$1.SD+ 11.2,91.2 6.2,91.2 6.2,78.2 5.2,77.2 E1.15
  Bottom 0.254: R8.2 8.6,77.4 8.4,77.2 5.2,77.2 E1.15
SPI_CLK
  Top 0.254: E2_EXT.5 57,25.4 55.8,24.2 55.8,20 55,19.2 51.4,19.2 51.4,26.8 52.2,27.6 52.2,51.6 52.8,52.2 52.8,64.2 54,65.4 57,65.4 57,64.4 E2.5
SPI_CS  (via drill 0.61)
  Top 0.254: v52.4,26.6 52.8,27 52.8,51.4 53.4,52 53.4,63 54.6,64.2 E2.6
  Bottom 0.254: v52.4,26.6 53.4,26.6 E2_EXT.6
SPI_MIS0
  Top 0.254: E2_EXT.4 54.8,23 55.2,23.4 55.2,24.4 55.8,25 55.8,60.8 54.8,61.8 E2.4
SPI_MOSI  (via drill 0.61)
  Top 0.254: v59.2,23 58.8,23.4 58.8,60.2 57.2,61.8 E2.3
  Bottom 0.254: v59.2,23 57.2,23 E2_EXT.3
UART_RX  (via drill 0.61)
  Top 0.254: v51.2,27.8 49.6,29.4 49.6,51.4 50.6,52.4 50.6,66 v51.8,67.2
  Bottom 0.254: v51.2,27.8 54.6,27.8 E2_EXT.8 | v51.8,67.2 52,67 54.6,67 E2.8
UART_TX  (via drill 0.61)
  Top 0.254: v51.2,29.2 51.6,29.6 51.6,51.8 51.8,52 51.8,65.2 53.4,66.8 53.4,67.2 54.2,68 57,68 57,67 E2.7
  Bottom 0.254: v51.2,29.2 53.4,29.2 53.6,29.4 55.6,29.4 57,28 E2_EXT.7

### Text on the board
tNames: Pitaya ADC/DAC | consorzio RFX Padova | 2018 | RePitaya interface | RF ADC isolated | G-Tronic Robotics | N | P | 1 | ing. Gottardo Phd 2017
bNames: DIO7_N M15 RESET- CH1 | DIO7_P M14 RESET+ CH1 | DIO6_N J16 CNVST- CH1 | DIO6_P J16 CNVST+ CH1 | DIO5_N L17 SCLK- CH1 | DIO5_P L16 SCLK+ CH1 | DIO4_N L15 DATA- CH1 | DIO4_P L14 DATA+ CH1 | DIO3_N K18 RESET- CH2 | DIO3_P K17 RESET+ CH2 | DIO2_N H18 CNVST- CH2 | DIO2_P J18 CNVST+ CH2 | DIO1_N H16 SCLK- CH2 | DIO1_P H16 SCLK+ CH2 | DIO0_N G18 DATA- CH2 | DIO0_P G17 DATA+ CH2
